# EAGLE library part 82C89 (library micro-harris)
MICROCONTROLLER/MEMORY DEVICE
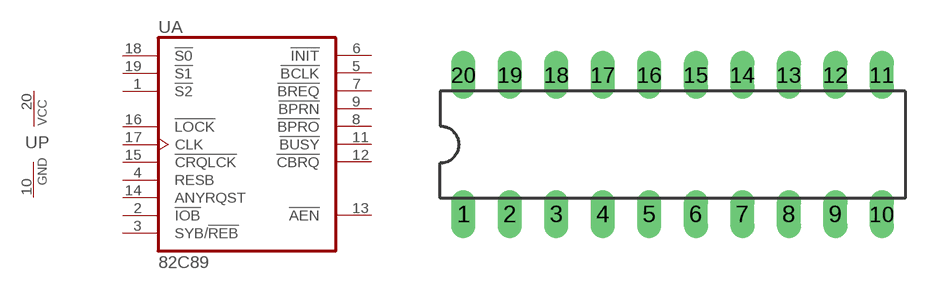
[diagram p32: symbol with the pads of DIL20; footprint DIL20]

Designator prefix U; gates A=82C89 P=PWRN

## 82C89 (MF: INTERSIL; MPN: CP82C89; OC_FARNELL: unknown; OC_NEWARK: 16F4897)  [DIL20]
1  A:!S2  in
2  A:!IOB  in
3  A:SYB/!REB  in
4  A:RESB  in
5  A:!BCLK  in
6  A:!INIT  in
7  A:!BREQ  out
8  A:!BPRO  out
9  A:!BPRN  in
10  P:GND  pwr
11  A:!BUSY
12  A:!CBRQ
13  A:!AEN  out
14  A:ANYRQST  in
15  A:!CRQLCK  in
16  A:!LOCK  in
17  A:CLK  in
18  A:!S0  in
19  A:!S1  in
20  P:VCC  pwr

## Footprint DIL20 (pad centres in mm)
Dual In Line Package
drill 0.813 long: 1 -11.43,-3.81; 2 -8.89,-3.81; 3 -6.35,-3.81; 4 -3.81,-3.81; 5 -1.27,-3.81; 6 1.27,-3.81; 7 3.81,-3.81; 8 6.35,-3.81; 9 8.89,-3.81; 10 11.43,-3.81; 11 11.43,3.81; 12 8.89,3.81; 13 6.35,3.81; 14 3.81,3.81; 15 1.27,3.81; 16 -1.27,3.81; 17 -3.81,3.81; 18 -6.35,3.81; 19 -8.89,3.81; 20 -11.43,3.81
